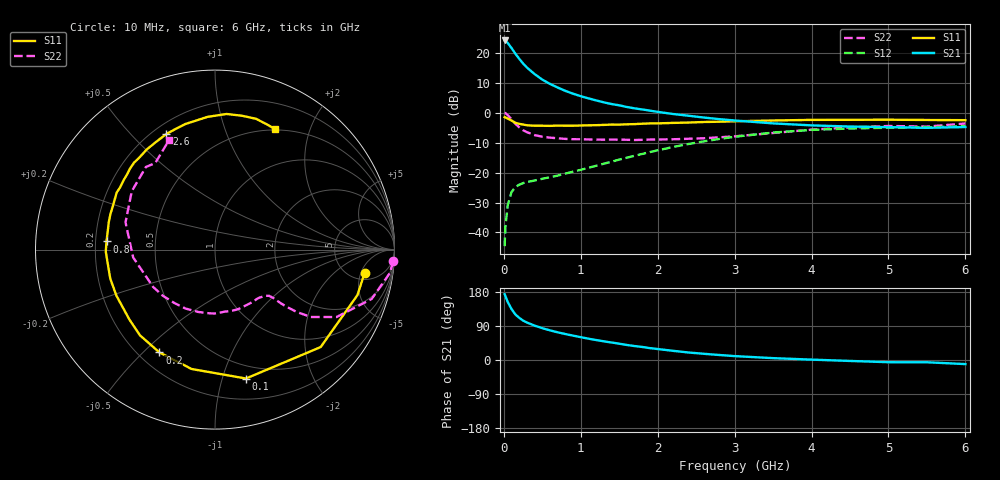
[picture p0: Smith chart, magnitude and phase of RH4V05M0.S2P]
! SIEMENS Small Signal Semiconductors
! BFR106
! Si NPN RF Bipolar Junction Transistor in SOT23
! VCE = 4 V  IC = 5 mA
! Common Emitter S-Parameters:  August  1996
# GHz  S  MA  R  50
!  f  S11  S21  S12  S22
! GHz  MAG  ANG  MAG  ANG  MAG  ANG  MAG  ANG
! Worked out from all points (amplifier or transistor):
!   36 points, 10 MHz to 6 GHz, reference 50 ohm
!   highest |S21| = 24.1 dB at 10 MHz (marker M1)
!   |S21| within 3 dB of that: start of sweep to 112.2 MHz
!   unconditionally stable (mu >= 1): 619.2 MHz to 1.894 GHz; 4.76 GHz to end of sweep
!   at 250 MHz: K = 0.50, MSG = 20.0 dB, |S12| = -23.5 dB
!   at 1.4 GHz: K = 1.14, MAG = 7.4 dB, |S12| = -16.4 dB
!   at 6 GHz: K = 1.02, MAG = -1.0 dB, |S12| = -4.5 dB
!   S11 on the Smith chart (normalised r, x): 10 MHz: 6.44, -5.82; 100 MHz: 0.38, -1.20; 200 MHz: 0.28, -0.56; 800 MHz: 0.25, +0.04; 2.6 GHz: 0.25, +0.63; 6 GHz: 0.49, +1.50
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0.01  0.8434 -8.9  16.08 173.6  0.0059 85.3  0.9945 -3.8
0.02  0.8332 -17.7  15.91 169.0  0.0122 81.2  0.9831 -7.6
0.05  0.8009 -42.7  14.63 153.3  0.0285 68.5  0.9151 -17.5
0.1  0.7386 -76.5  12.01 134.4  0.0474 54.3  0.7749 -29.0
0.15  0.6778 -101.1  9.648 120.2  0.0572 45.6  0.653 -35.1
0.2  0.6513 -118.4  7.948 111.3  0.0627 41.3  0.5711 -37.4
0.25  0.6346 -131.2  6.621 104.0  0.0667 38.7  0.5101 -38.6
0.3  0.6161 -140.6  5.677 98.9  0.0693 38.6  0.4732 -39.2
0.4  0.6063 -155.0  4.413 90.7  0.0737 39.1  0.4225 -39.7
0.5  0.6055 -164.5  3.567 84.0  0.0787 41.5  0.3965 -40.5
0.6  0.6027 -172.6  3.023 78.2  0.0837 44.0  0.3833 -42.2
0.8  0.6061 175.7  2.313 68.5  0.0961 49.9  0.365 -47.0
1.1  0.6154 161.2  1.735 56.3  0.1204 57.0  0.3575 -56.5
1.3  0.6251 153.2  1.489 49.3  0.1407 60.0  0.3546 -63.8
1.6  0.6398 142.5  1.244 39.7  0.1773 62.1  0.3531 -76.4
2.2  0.6753 124.2  0.951 24.2  0.2673 59.3  0.3598 -105.1
2.6  0.6989 112.8  0.83 16.4  0.332 53.8  0.3738 -127.0
3.5  0.7404 93.3  0.663 4.9  0.466 37.1  0.458 -174.5
4.5  0.7608 78.5  0.587 -2.5  0.5437 17.6  0.5665 144.9
5  0.7637 72.7  0.574 -5.8  0.5607 9.5  0.6 129.9
5.5  0.7553 67.4  0.559 -6.0  0.5695 5.5  0.586 124.6
6  0.75 63.6  0.576 -10.8  0.5962 -2.4  0.6605 112.9
